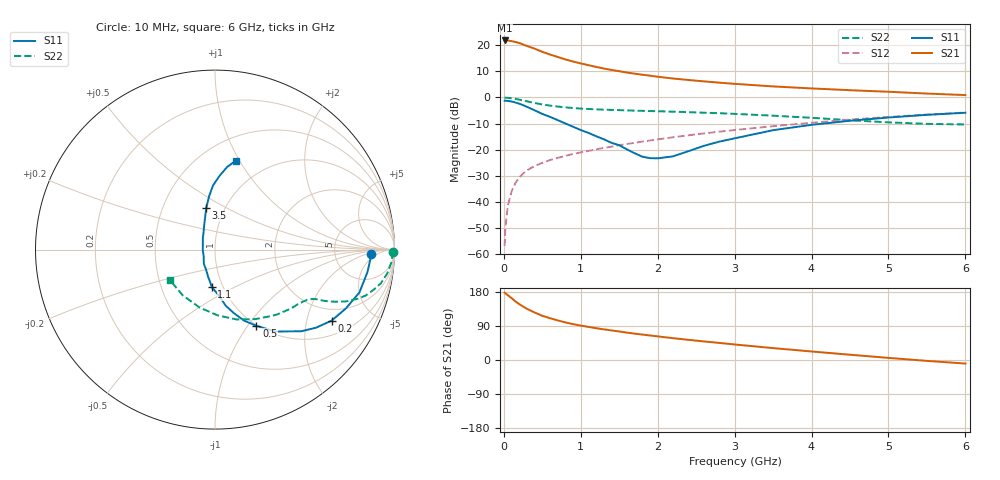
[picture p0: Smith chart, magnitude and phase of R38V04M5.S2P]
! SIEMENS Small Signal Semiconductors
! BFR181
! Si NPN RF Bipolar Junction Transistor in SOT23
! VCE = 8 V  IC = 4.5 mA
! Common Emitter S-Parameters:  May  1996
# GHz  S  MA  R  50
!  f  S11  S21  S12  S22
! GHz  MAG  ANG  MAG  ANG  MAG  ANG  MAG  ANG
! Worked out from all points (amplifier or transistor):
!   36 points, 10 MHz to 6 GHz, reference 50 ohm
!   highest |S21| = 21.9 dB at 10 MHz (marker M1)
!   |S21| within 3 dB of that: start of sweep to 385.7 MHz
!   unconditionally stable (mu >= 1): 1.243 GHz to 3.143 GHz
!   at 250 MHz: K = 0.38, MSG = 24.8 dB, |S12| = -29.2 dB
!   at 1.4 GHz: K = 1.03, MAG = 13.7 dB, |S12| = -18.9 dB
!   at 6 GHz: K = 0.86, MSG = 3.4 dB, |S12| = -5.8 dB
!   S11 on the Smith chart (normalised r, x): 10 MHz: 14, -3; 200 MHz: 1.51, -2.84; 500 MHz: 0.99, -1.10; 1.1 GHz: 0.88, -0.39; 3.5 GHz: 0.82, +0.40; 6 GHz: 0.72, +0.97
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0.01  0.869 -1.8  12.44 177.7  0.0014 104.2  0.9923 -0.7
0.02  0.868 -3.2  12.31 175.9  0.0032 83.4  0.9892 -1.7
0.05  0.8589 -8.3  12.41 171.3  0.0081 84.9  0.9862 -4.0
0.1  0.8394 -16.5  12.1 163.4  0.0157 81.0  0.9691 -7.9
0.15  0.7995 -24.2  11.62 154.6  0.0227 76.0  0.9427 -11.5
0.2  0.761 -31.3  11.13 147.6  0.0292 73.9  0.9106 -14.3
0.25  0.7116 -37.7  10.43 141.1  0.0345 70.6  0.8783 -16.9
0.3  0.6621 -43.4  9.763 135.1  0.0398 68.7  0.8458 -18.8
0.4  0.5681 -53.5  8.658 125.4  0.0484 65.7  0.7845 -21.6
0.5  0.4831 -61.5  7.527 116.6  0.0557 63.9  0.7343 -23.3
0.6  0.426 -67.9  6.681 110.3  0.063 62.8  0.6989 -24.4
0.8  0.3179 -79.2  5.386 99.2  0.076 62.2  0.6467 -25.7
0.9  0.2741 -83.1  4.902 94.6  0.0824 62.7  0.6277 -26.1
1.1  0.2089 -95.1  4.171 87.4  0.0943 63.0  0.6017 -27.3
1.3  0.1576 -104.0  3.598 80.9  0.1077 63.2  0.5842 -28.6
1.6  0.1009 -127.7  3.012 72.2  0.128 62.8  0.566 -31.2
1.9  0.0684 -164.8  2.624 64.7  0.1497 62.7  0.5489 -34.2
2.2  0.0742 156.1  2.313 57.6  0.1725 61.6  0.5343 -37.9
3.5  0.2357 102.0  1.631 31.4  0.2812 53.3  0.4479 -59.8
4.5  0.3576 91.8  1.38 13.9  0.3761 43.6  0.3664 -87.9
5.5  0.4648 81.7  1.19 -2.3  0.4702 31.5  0.3119 -125.4
6  0.5095 76.8  1.112 -9.4  0.5141 24.6  0.3034 -146.4
